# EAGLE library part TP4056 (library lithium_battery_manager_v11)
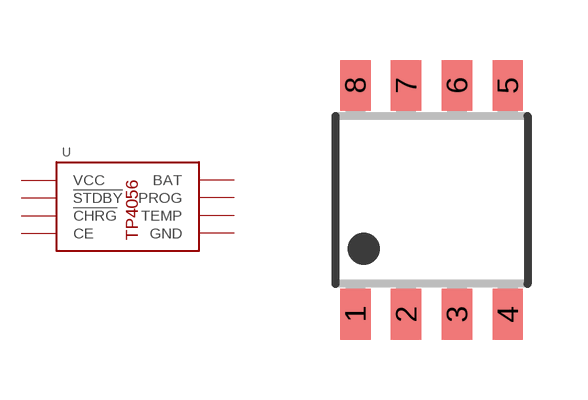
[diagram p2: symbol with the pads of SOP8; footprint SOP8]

Designator prefix -

## TP4056  [SOP8]
1  TEMP
2  PROG
3  GND
4  VCC
5  BAT
6  !STDBY
7  !CHRG
8  CE

## Footprint SOP8 (pad centres in mm)
Small Outline Package 8 8P2S-A Plastic 8pin 225mil SOP Source: Mitsubishi M5218AL/P/FP
smd 0.76 x 1.27: 1 -1.905,-2.86; 2 -0.635,-2.86; 3 0.635,-2.86; 4 1.905,-2.86; 5 1.905,2.86; 6 0.635,2.86; 7 -0.635,2.86; 8 -1.905,2.86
